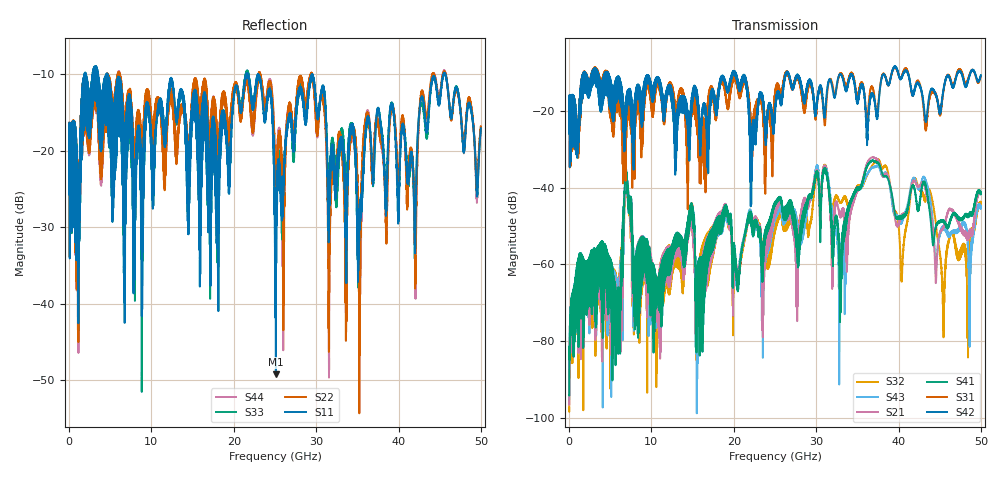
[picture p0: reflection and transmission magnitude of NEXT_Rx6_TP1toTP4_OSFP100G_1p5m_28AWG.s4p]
! Touchstone data
! Created: 27-Feb-2019 by IdEM 12 (12.1.0)
! COMMENTS
!  Created Wed Feb 27 09:43:39 2019
!  64 Port Network Data from SP1.SP block
!  freq  magS1_1  angS1_1  magS1_2  angS1_2  magS1_3  angS1_3  magS1_4  angS1_4
!  magS1_5  angS1_5  magS1_6  angS1_6  magS1_7  angS1_7  magS1_8  angS1_8
!  magS1_9  angS1_9  magS1_10  angS1_10  magS1_11  angS1_11  magS1_12  angS1_12
!  magS1_13  angS1_13  magS1_14  angS1_14  magS1_15  angS1_15  magS1_16  angS1_16
!  magS1_17  angS1_17  magS1_18  angS1_18  magS1_19  angS1_19  magS1_20  angS1_20
!  magS1_21  angS1_21  magS1_22  angS1_22  magS1_23  angS1_23  magS1_24  angS1_24
!  magS1_25  angS1_25  magS1_26  angS1_26  magS1_27  angS1_27  magS1_28  angS1_28
!  magS1_29  angS1_29  magS1_30  angS1_30  magS1_31  angS1_31  magS1_32  angS1_32
!  magS1_33  angS1_33  magS1_34  angS1_34  magS1_35  angS1_35  magS1_36  angS1_36
!  magS1_37  angS1_37  magS1_38  angS1_38  magS1_39  angS1_39  magS1_40  angS1_40
!  magS1_41  angS1_41  magS1_42  angS1_42  magS1_43  angS1_43  magS1_44  angS1_44
!  magS1_45  angS1_45  magS1_46  angS1_46  magS1_47  angS1_47  magS1_48  angS1_48
!  magS1_49  angS1_49  magS1_50  angS1_50  magS1_51  angS1_51  magS1_52  angS1_52
!  magS1_53  angS1_53  magS1_54  angS1_54  magS1_55  angS1_55  magS1_56  angS1_56
!  magS1_57  angS1_57  magS1_58  angS1_58  magS1_59  angS1_59  magS1_60  angS1_60
!  magS1_61  angS1_61  magS1_62  angS1_62  magS1_63  angS1_63  magS1_64  angS1_64
!  magS2_1  angS2_1  magS2_2  angS2_2  magS2_3  angS2_3  magS2_4  angS2_4
!  magS2_5  angS2_5  magS2_6  angS2_6  magS2_7  angS2_7  magS2_8  angS2_8
!  magS2_9  angS2_9  magS2_10  angS2_10  magS2_11  angS2_11  magS2_12  angS2_12
!  magS2_13  angS2_13  magS2_14  angS2_14  magS2_15  angS2_15  magS2_16  angS2_16
!  magS2_17  angS2_17  magS2_18  angS2_18  magS2_19  angS2_19  magS2_20  angS2_20
!  magS2_21  angS2_21  magS2_22  angS2_22  magS2_23  angS2_23  magS2_24  angS2_24
!  magS2_25  angS2_25  magS2_26  angS2_26  magS2_27  angS2_27  magS2_28  angS2_28
!  magS2_29  angS2_29  magS2_30  angS2_30  magS2_31  angS2_31  magS2_32  angS2_32
!  magS2_33  angS2_33  magS2_34  angS2_34  magS2_35  angS2_35  magS2_36  angS2_36
!  magS2_37  angS2_37  magS2_38  angS2_38  magS2_39  angS2_39  magS2_40  angS2_40
!  magS2_41  angS2_41  magS2_42  angS2_42  magS2_43  angS2_43  magS2_44  angS2_44
!  magS2_45  angS2_45  magS2_46  angS2_46  magS2_47  angS2_47  magS2_48  angS2_48
!  magS2_49  angS2_49  magS2_50  angS2_50  magS2_51  angS2_51  magS2_52  angS2_52
!  magS2_53  angS2_53  magS2_54  angS2_54  magS2_55  angS2_55  magS2_56  angS2_56
!  magS2_57  angS2_57  magS2_58  angS2_58  magS2_59  angS2_59  magS2_60  angS2_60
!  magS2_61  angS2_61  magS2_62  angS2_62  magS2_63  angS2_63  magS2_64  angS2_64
!  magS3_1  angS3_1  magS3_2  angS3_2  magS3_3  angS3_3  magS3_4  angS3_4
!  magS3_5  angS3_5  magS3_6  angS3_6  magS3_7  angS3_7  magS3_8  angS3_8
!  magS3_9  angS3_9  magS3_10  angS3_10  magS3_11  angS3_11  magS3_12  angS3_12
!  magS3_13  angS3_13  magS3_14  angS3_14  magS3_15  angS3_15  magS3_16  angS3_16
!  magS3_17  angS3_17  magS3_18  angS3_18  magS3_19  angS3_19  magS3_20  angS3_20
!  magS3_21  angS3_21  magS3_22  angS3_22  magS3_23  angS3_23  magS3_24  angS3_24
!  magS3_25  angS3_25  magS3_26  angS3_26  magS3_27  angS3_27  magS3_28  angS3_28
!  magS3_29  angS3_29  magS3_30  angS3_30  magS3_31  angS3_31  magS3_32  angS3_32
!  magS3_33  angS3_33  magS3_34  angS3_34  magS3_35  angS3_35  magS3_36  angS3_36
!  magS3_37  angS3_37  magS3_38  angS3_38  magS3_39  angS3_39  magS3_40  angS3_40
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# Hz S MA R 50
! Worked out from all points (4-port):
!   5000 points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, 10 MHz to 50 GHz, reference 50 ohm
!   strongest paths, dB at 10 MHz, 12.51 GHz, 25.01 GHz, 37.51 GHz, 50 GHz:
!     S42: -19.6, -16.4, -19.1, -20.0, -10.6
!     S31: -19.6, -14.0, -15.9, -19.1, -11.0
!     S41: -94.1, -56.5, -43.8, -33.5, -41.6
!     S21: -96.4, -56.7, -45.5, -32.8, -41.3
!     S43: -95.5, -56.9, -47.1, -34.3, -45.0
!     S32: -97.5, -56.9, -49.1, -32.7, -43.9
!   lowest |S11| = -49.2 dB at 25.11 GHz (marker M1), VSWR 1.01, Z = 50.3 + j0.113 ohm
!   |S11| at or under -10 dB: 4.66 GHz to 21.51 GHz (16.85 GHz wide, 129 % of centre); 22.94 GHz to 45.47 GHz (22.53 GHz wide, 65.9 % of centre); 45.68 GHz to end of sweep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
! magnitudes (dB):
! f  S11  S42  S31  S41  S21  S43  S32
! 10 MHz  -19.2  -19.6  -19.6  -94.1  -96.4  -95.5  -97.5
! 5.95 GHz  -11.6  -11.3  -12.2  -66.2  -67.0  -64.8  -66.3
! 6.97 GHz  -16.0  -18.0  -19.8  -36.4  -37.0  -37.4  -38.0
! 10.66 GHz  -15.6  -11.8  -13.2  -69.1  -74.7  -74.0  -69.5
! 25.11 GHz  -49.2  -17.2  -14.8  -43.5  -45.0  -46.7  -48.7
! 45.42 GHz  -10.2  -15.0  -15.4  -48.8  -50.4  -50.2  -75.7
! 50 GHz  -17.1  -10.6  -11.0  -41.6  -41.3  -45.0  -43.9
